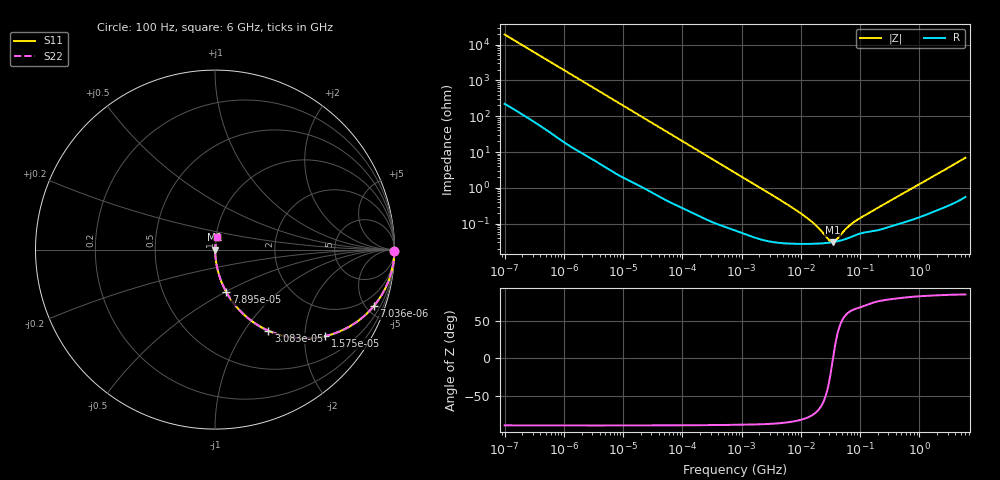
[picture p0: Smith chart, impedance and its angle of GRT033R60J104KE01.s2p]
!Murata Part Number: GRT033R60J104KE01
!These Parameters are Measured in Series Mode Connection
!Data Generated on Jun 19, 2026
!  o--ll--o
!Port1  Port2
!  o------o
!Operation Temp=25[degC], DC Bias Voltage=0[V]
!Freq. Start=100[Hz] Stop=6[GHz] 401[Steps]
# Hz S RI R 50
!Freq.(Hz) S11(Real) S11(Imag) S21(Real) S21(Imag) S12(Real) S12(Imag) S22(Real) S22(Imag)
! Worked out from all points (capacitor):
!   401 points, 100 Hz to 6 GHz, reference 50 ohm
!   read as one part in series: C = 82.4 nF near 109 Hz
!   lowest |Z| = 30.3 mohm at 34.83 MHz (marker M1)
!   series resonance near 34.88 MHz, so ESL is about 250 pH
!   S11 on the Smith chart (normalised r, x): 100 Hz: open; 7.036 kHz: 1.05, -5.63; 15.75 kHz: 1.03, -2.53; 30.83 kHz: 1.01, -1.30; 78.95 kHz: 1.01, -0.51; 6 GHz: 1.01, +0.14
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100  0.9999 -0.00519  8.67e-05 0.00519  8.67e-05 0.00519  0.9999 -0.00519
627  0.9986 -0.032  0.00136 0.032  0.00136 0.032  0.9986 -0.032
2008  0.9887 -0.1009  0.0113 0.1009  0.0113 0.1009  0.9887 -0.1009
4111  0.9567 -0.1988  0.0433 0.1988  0.0433 0.1988  0.9567 -0.1988
7036  0.8856 -0.3136  0.1144 0.3136  0.1144 0.3136  0.8856 -0.3136
10527  0.7781 -0.4106  0.2219 0.4106  0.2219 0.4106  0.7781 -0.4106
15752  0.6135 -0.4817  0.3865 0.4817  0.3865 0.4817  0.6135 -0.4817
21550  0.4616 -0.4931  0.5384 0.4931  0.5384 0.4931  0.4616 -0.4931
30832  0.298 -0.4518  0.702 0.4518  0.702 0.4518  0.298 -0.4518
40335  0.2005 -0.3947  0.7995 0.3947  0.7995 0.3947  0.2005 -0.3947
78952  0.0636 -0.2378  0.9364 0.2378  0.9364 0.2378  0.0636 -0.2378
211427  0.0106 -0.0948  0.9894 0.0948  0.9894 0.0948  0.0106 -0.0948
774597  0.00134 -0.0264  0.9987 0.0264  0.9987 0.0264  0.00134 -0.0264
6353432  0.000286 -0.00317  0.9997 0.00317  0.9997 0.00317  0.000286 -0.00317
1.555665e7  0.000273 -0.00107  0.9997 0.00107  0.9997 0.00107  0.000273 -0.00107
3.045065e7  0.000293 -0.000161  0.9997 0.000161  0.9997 0.000161  0.000293 -0.000161
3.482834e7  0.000303 -1.8e-06  0.9997 1.8e-06  0.9997 1.8e-06  0.000303 -1.8e-06
3.983537e7  0.000315 0.000157  0.9997 -0.000157  0.9997 -0.000157  0.000315 0.000157
5.960426e7  0.000381 0.000644  0.9996 -0.000644  0.9996 -0.000644  0.000381 0.000644
8.154455e7  0.000467 0.00105  0.9995 -0.00105  0.9995 -0.00105  0.000467 0.00105
3.124326e8  0.000827 0.00414  0.9992 -0.00414  0.9992 -0.00414  0.000827 0.00414
6e9  0.0102 0.0679  0.9898 -0.0679  0.9898 -0.0679  0.0102 0.0679
